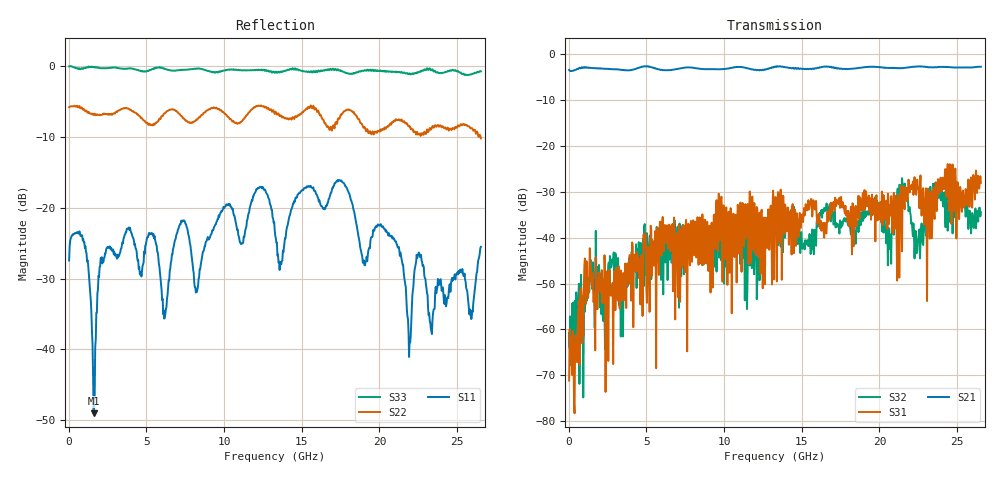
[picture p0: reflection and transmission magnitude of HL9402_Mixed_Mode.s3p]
! HYPERLABS, INC. 03/12/2021
! MIXED MODE  S-PARAMETERS
! CALCULATED FROM A MEASURED DATA S3P FILE
# GHZ S RI R 50.0
! FREQ.GHZ S11 SSD12 SSC12
! SDS21 SDD22 SDC22
! SCS21 SCD22 SCC22
!; PortSelection: Port_123
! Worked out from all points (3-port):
!   758 points, 35 MHz to 26.53 GHz, reference 50 ohm
!   strongest paths, dB at 35 MHz, 6.65 GHz, 13.3 GHz, 19.91 GHz, 26.53 GHz:
!     S21: -3.4, -3.4, -2.7, -2.8, -2.7
!     S31: -71.2, -37.2, -31.1, -32.6, -28.0
!     S32: -60.8, -45.2, -37.4, -33.9, -34.5
!   lowest |S11| = -49.1 dB at 1.61 GHz (marker M1), VSWR 1.01, Z = 49.8 - j0.302 ohm
!   |S11| at or under -10 dB: start of sweep to end of sweep
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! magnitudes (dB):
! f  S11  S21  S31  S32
! 35 MHz  -27.5  -3.4  -71.2  -60.8
! 1.05 GHz  -25.7  -2.9  -44.5  -56.1
! 1.61 GHz  -49.1  -3.0  -54.1  -50.9
! 2.03 GHz  -28.3  -3.0  -51.7  -55.2
! 3.85 GHz  -23.0  -3.5  -48.8  -47.9
! 6.195 GHz  -35.4  -3.5  -37.2  -40.7
! 13.3 GHz  -23.9  -2.7  -31.1  -37.4
! 17.61 GHz  -16.4  -3.2  -32.9  -37.4
! 21.95 GHz  -38.6  -2.9  -30.1  -33.4
! 26.53 GHz  -25.5  -2.7  -28.0  -34.5
